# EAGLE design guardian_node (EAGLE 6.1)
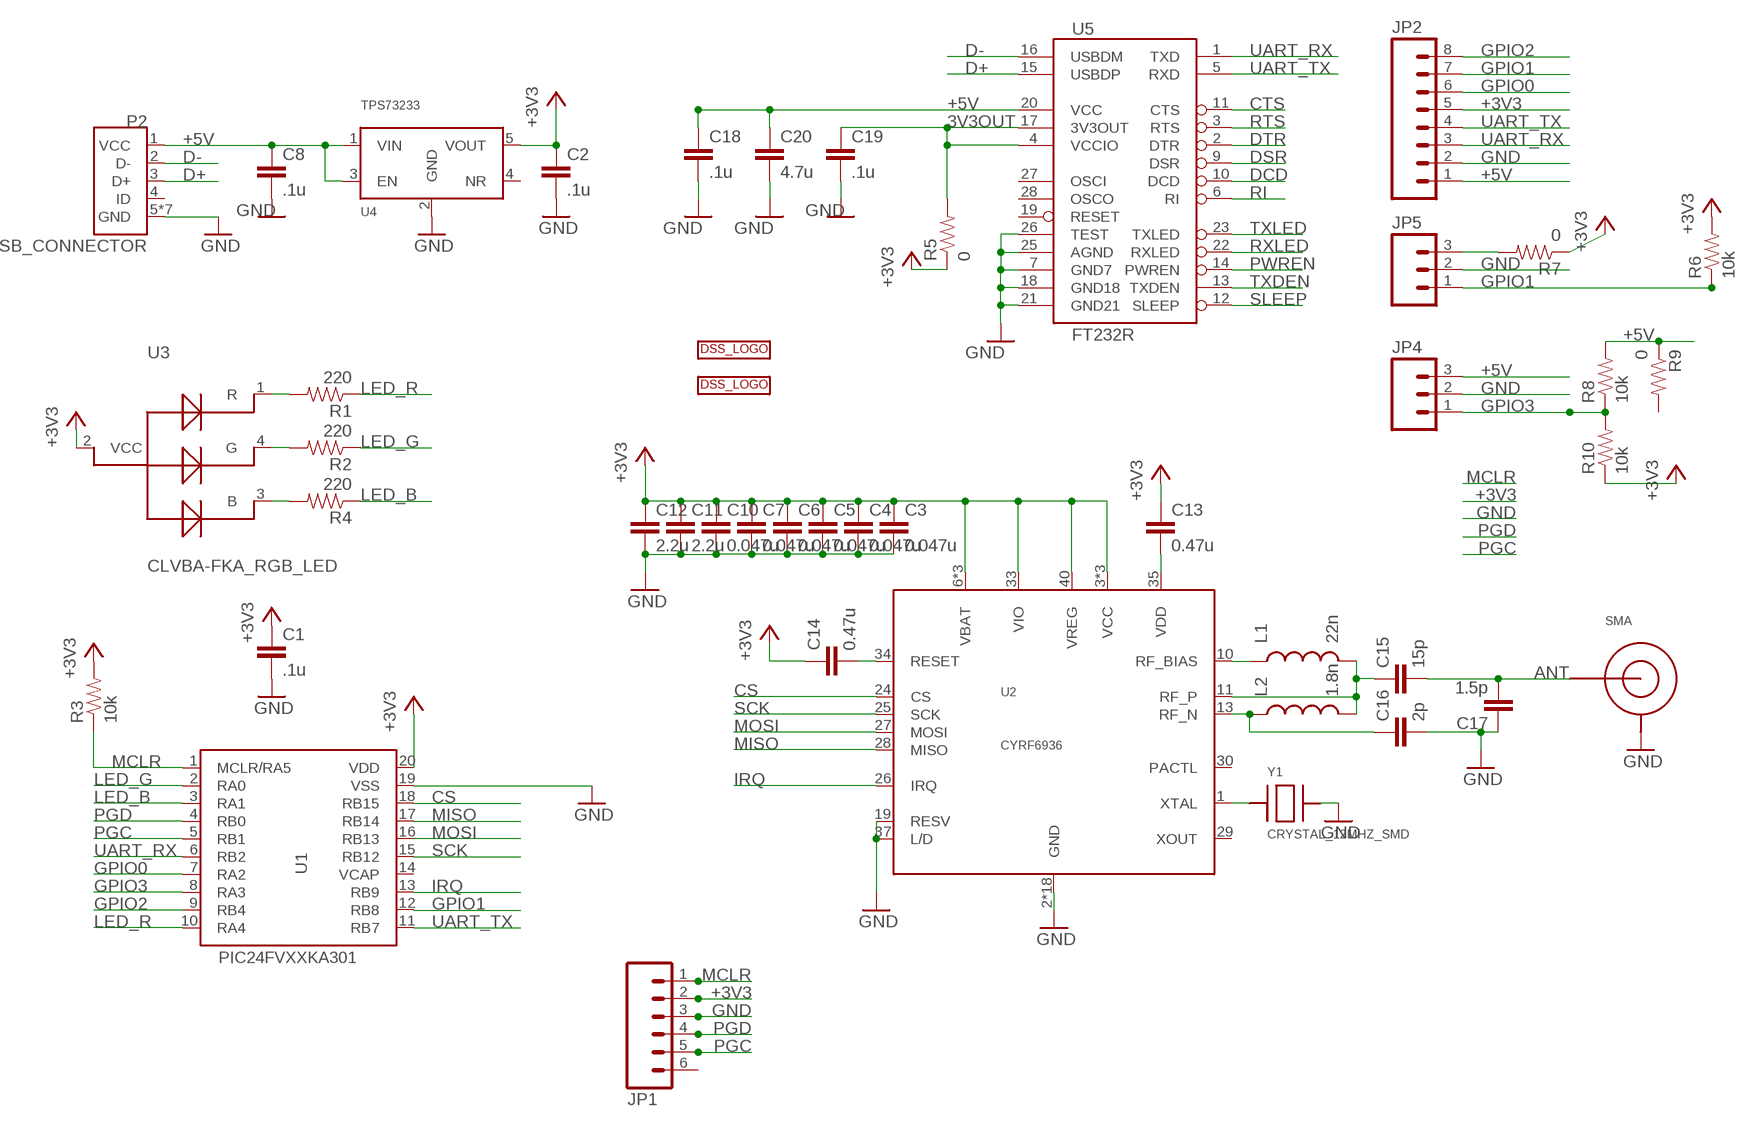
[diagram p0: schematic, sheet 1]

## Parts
C1  .1u  CAP0603-CAP  [0603-CAP]
C2  .1u  CAP0603-CAP  [0603-CAP]
C3  0.047u  CAP0402-CAP  [0402-CAP]
C4  0.047u  CAP0402-CAP  [0402-CAP]
C5  0.047u  CAP0402-CAP  [0402-CAP]
C6  0.047u  CAP0402-CAP  [0402-CAP]
C7  0.047u  CAP0402-CAP  [0402-CAP]
C8  .1u  CAP0603-CAP  [0603-CAP]
C10  0.047u  CAP0402-CAP  [0402-CAP]
C11  2.2u  CAP0402-CAP  [0402-CAP]
C12  2.2u  CAP0402-CAP  [0402-CAP]
C13  0.47u  CAP0402-CAP  [0402-CAP]
C14  0.47u  CAP0402-CAP  [0402-CAP]
C15  15p  CAP0402-CAP  [0402-CAP]
C16  2p  CAP0402-CAP  [0402-CAP]
C17  1.5p  CAP0402-CAP  [0402-CAP]
C18  .1u  CAP0603-CAP  [0603-CAP]
C19  .1u  CAP0603-CAP  [0603-CAP]
C20  4.7u  CAP0603-CAP  [0603-CAP]
JP1  M06SIP  [1X06]
JP2  M081X08  [1X08]
JP4  M03PTH  [1X03]
JP5  M03PTH  [1X03]
L1  22n  INDUCTOR0603  [0603]
L2  1.8n  INDUCTOR0402  [C0402]
P2  USB_CONNECTOR  [USB_MICRO]
R1  220  RESISTOR0402-RES  [0402-RES]
R2  220  RESISTOR0402-RES  [0402-RES]
R3  10k  RESISTOR0603-RES  [0603-RES]
R4  220  RESISTOR0402-RES  [0402-RES]
R5  0  RESISTOR0603-RES  [0603-RES]
R6  10k  RESISTOR0603-RES  [0603-RES]
R7  0  RESISTOR0603-RES  [0603-RES]
R8  10k  RESISTOR0603-RES  [0603-RES]
R9  0  RESISTOR0603-RES  [0603-RES]
R10  10k  RESISTOR0603-RES  [0603-RES]
SMA  SMA_PTH  [SMA_PTH]
U1  PIC24FVXXKA301  [SSOP20]
U2  CYRF6936  [QFN40-6X6]
U3  CLVBA-FKA_RGB_LED  [PLCC-4]
U4  TPS73233  [SOT23-5]
U5  FT232R  FT232RLSSOP  [SSOP28DB]
U$1  DSSBOTTOM  [DSS_BOT]
U$2  DSSTOP  [DSS]
Y1  CRYSTAL_12MHZ_SMD  [SMD-4_5X3.2MM]

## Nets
3V3OUT: C19.1 R5.2 U5.4(VCCIO) U5.17(3V3OUT)
+3V3: C1.1 C2.1 C3.1 C4.1 C5.1 C6.1 C7.1 C10.1 C11.1 C12.1 C13.1 C14.1 JP1.2 JP2.5 R3.2 R5.1 R6.2 R7.1 R10.1 U1.20(VDD) U2.3(VCC) U2.6(VBAT) U2.7(VCC) U2.8(VBAT) U2.16(VCC) U2.33(VIO) U2.38(VBAT) U2.40(VREG) U3.2(VCC) U4.5(VOUT)
+5V: C8.1 C18.1 C20.1 JP2.1 JP4.3 P2.1(VCC) R8.2 R9.1 U4.1(VIN) U4.3(EN) U5.20(VCC)
ANT: C15.2 C17.2 SMA.PIN(CENTER)
CS: U1.18(RB15) U2.24(CS)
CTS: U5.11(CTS)
D+: P2.3(D+) U5.15(USBDP)
D-: P2.2(D-) U5.16(USBDM)
DCD: U5.10(DCD)
DSR: U5.9(DSR)
DTR: U5.2(DTR)
GND: C1.2 C2.2 C3.2 C4.2 C5.2 C6.2 C7.2 C8.2 C10.2 C11.2 C12.2 C16.2 C17.1 C18.2 C19.2 C20.2 JP1.3 JP2.2 JP4.2 JP5.2 P2.5(GND) P2.GND1(GND) P2.GND2(GND) P2.GND3(GND) P2.GND4(GND) P2.GND5(GND) P2.GND6(GND) SMA.GND1(SHIELD) SMA.GND2(SHIELD) SMA.GND3(SHIELD) SMA.GND4(SHIELD) U1.19(VSS) U2.2(GND) U2.4(GND) U2.5(GND) U2.9(GND) U2.12(GND) U2.14(GND) U2.15(GND) U2.17(GND) U2.18(GND) U2.19(RESV) U2.20(GND) U2.21(GND) U2.22(GND) U2.23(GND) U2.31(GND) U2.32(GND) U2.36(GND) U2.37(L/D) U2.39(GND) U2.EXP(GND) U4.2(GND) U5.7(GND7) U5.18(GND18) U5.21(GND21) U5.25(AGND) U5.26(TEST) Y1.P$3
GPIO0: JP2.6 U1.7(RA2)
GPIO1: JP2.7 JP5.1 R6.1 U1.12(RB8)
GPIO2: JP2.8 U1.9(RB4)
GPIO3: JP4.1 R8.1 R10.2 U1.8(RA3)
IRQ: U1.13(RB9) U2.26(IRQ)
LED_B: R4.1 U1.3(RA1)
LED_G: R2.1 U1.2(RA0)
LED_R: R1.1 U1.10(RA4)
MCLR: JP1.1 R3.1 U1.1(MCLR/RA5)
MISO: U1.17(RB14) U2.28(MISO)
MOSI: U1.16(RB13) U2.27(MOSI)
N$1: R1.2 U3.1(R)
N$2: R2.2 U3.4(G)
N$3: R4.2 U3.3(B)
N$4: JP5.3 R7.2
N$5: L1.1 U2.10(RF_BIAS)
N$6: C15.1 L1.2 L2.2 U2.11(RF_P)
N$7: C13.2 U2.35(VDD)
N$8: C14.2 U2.34(RESET)
N$9: C16.1 L2.1 U2.13(RF_N)
N$10: U2.1(XTAL) Y1.P$1
PGC: JP1.5 U1.5(RB1)
PGD: JP1.4 U1.4(RB0)
PWREN: U5.14(PWREN)
RI: U5.6(RI)
RTS: U5.3(RTS)
RXLED: U5.22(RXLED)
SCK: U1.15(RB12) U2.25(SCK)
SLEEP: U5.12(SLEEP)
TXDEN: U5.13(TXDEN)
TXLED: U5.23(TXLED)
UART_RX: JP2.3 U1.6(RB2) U5.1(TXD)
UART_TX: JP2.4 U1.11(RB7) U5.5(RXD)
Unconnected: JP1.6 P2.4(ID) R9.2 U1.14(VCAP) U2.29(XOUT) U2.30(PACTL) U4.4(NR) U5.19(RESET) U5.27(OSCI) U5.28(OSCO)

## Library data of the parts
C1-C8 C10-C20 = SparkFun-Passives:CAP: Capacitor
JP1 = SparkFun-Connectors:M06: Header 6 Standard 6-pin 0.1" header. Use with straight break away headers (SKU : PRT-00116), right angle break away headers (PRT-00553), swiss pins (PRT-00743), machine pins (PRT-00117), and female headers (PRT-00115). Molex polarized connector foot print use with SKU : PRT-08094 with associated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
JP2 = SparkFun-Connectors:M08: Header 8 Standard 8-pin 0.1" header. Use with straight break away headers (SKU : PRT-00116), right angle break away headers (PRT-00553), swiss pins (PRT-00743), machine pins (PRT-00117), and female headers (PRT-00115).
JP4 JP5 = SparkFun-Connectors:M03: Header 3 Standard 3-pin 0.1" header. Use with straight break away headers (SKU : PRT-00116), right angle break away headers (PRT-00553), swiss pins (PRT-00743), machine pins (PRT-00117), and female headers (PRT-00115). Molex polarized connector foot print use with SKU : PRT-08232 with associated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
L1 L2 = SparkFun-Passives:INDUCTOR: Inductors
P2 = DSS:USB_CONNECTOR: USB Connector http://www.digikey.com/product-detail/en/10118192-0001LF/609-4613-1-ND/2785378
R1-R10 = SparkFun-Passives:RESISTOR: Resistor
SMA = DSS:SMA_PTH: SMA through-hole
U1 = DSS:PIC24FVXXKA301: PIC24FVXXKA301
U2 = DSS:CYRF6936: Cypress CYRF6936 2.4GHz DSSS radio. All N/C pins and the exposed pad are tied to ground.
U3 = DSS:CLVBA-FKA_RGB_LED
U4 = DSS:TPS73233: TI TPS73233 - fixed output http://www.ti.com/product/tps73233
U5 = SparkFun:FT232RL: USB UART FT232RL 4th Generation USB UART (USB <-> Serial) Controller. Spark Fun Electronics SKU : COM-00650
U$1 U$2 = DSS:DSS: DSS LOGO
Y1 = DSS:CRYSTAL_12MHZ_SMD: 12MHz crystal, SMD

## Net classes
2 VCC: width 0.406 mm, clearance 0.381 mm

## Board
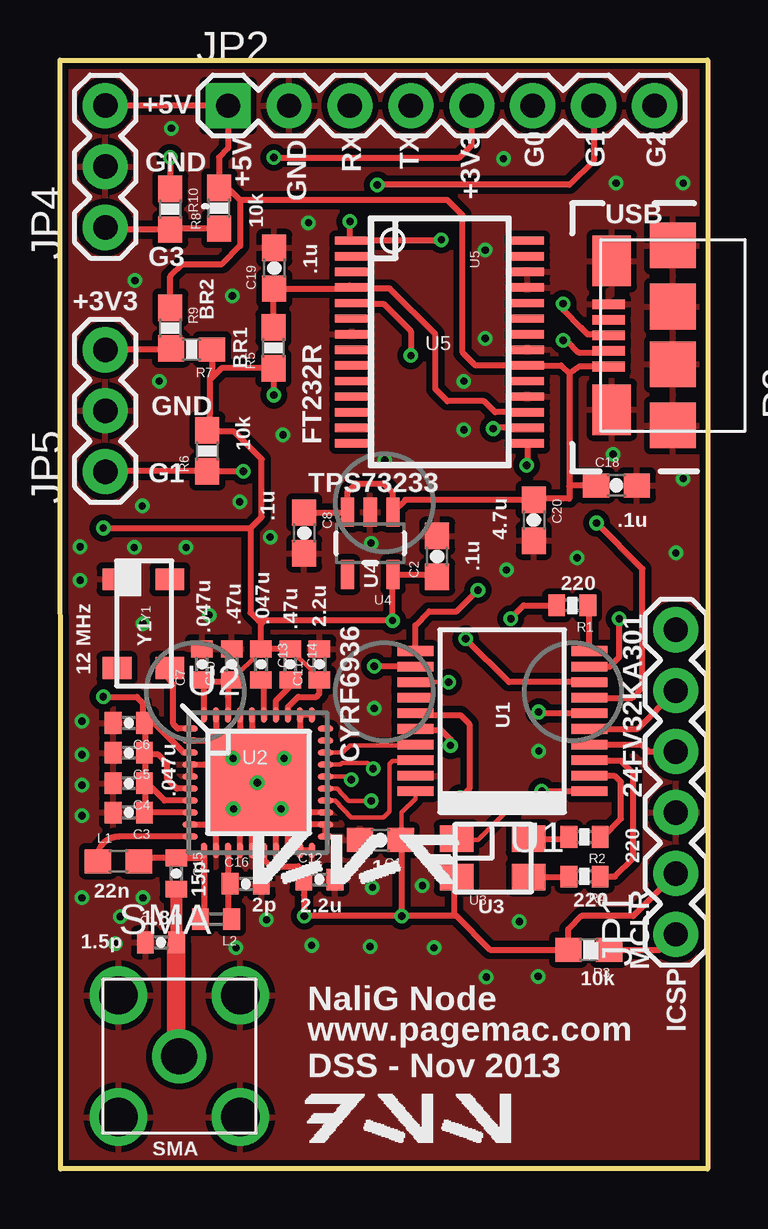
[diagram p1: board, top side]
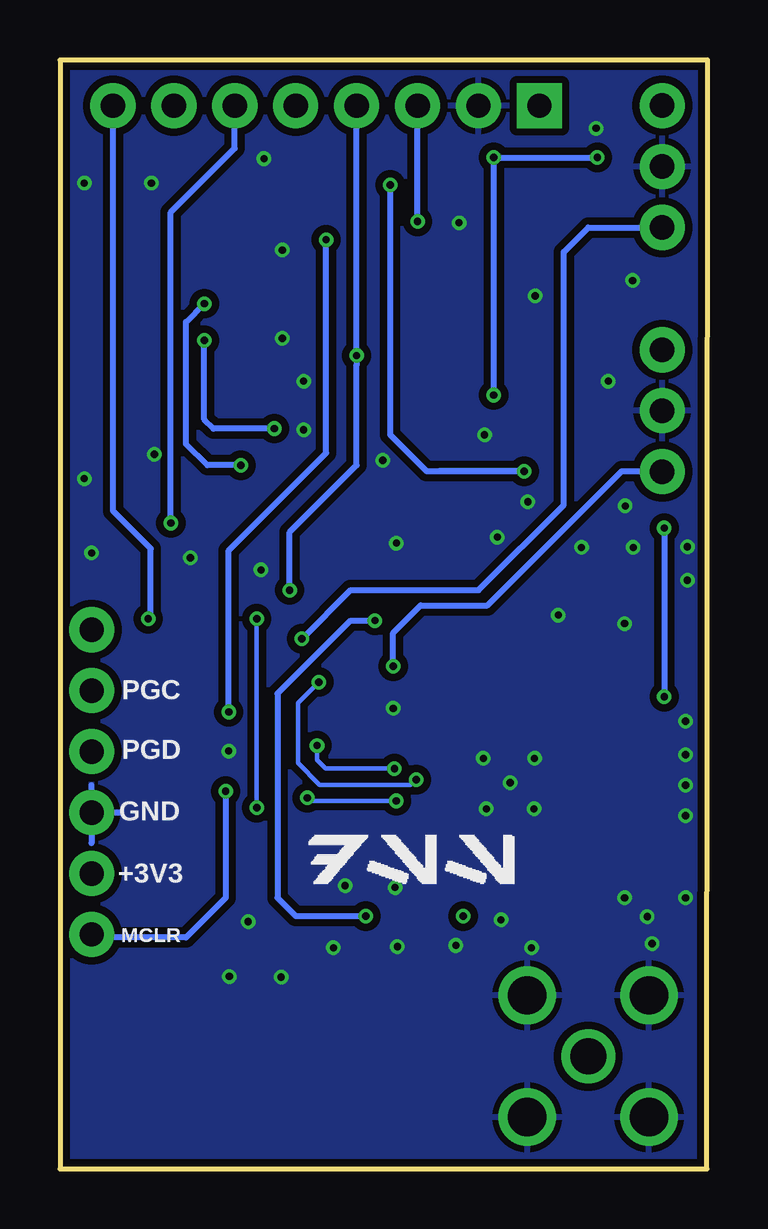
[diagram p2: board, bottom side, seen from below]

Size 27 x 46.23 mm. Coordinates in mm from the lower left corner, seen from the top.
Outline: 0,46.23 27,46.23 27,0 0.03,0 0,46.23
Copper layers (1*16): Top 0.035mm / dielectric 1.5mm / Bottom 0.035mm
Design rules: minimum track width 6mil, minimum drill 12mil, track to track 6mil, track to pad 6mil, pad to pad 6mil, via to via 6mil, smd to smd 0mil, copper to edge 10mil, drill to drill 10mil, minimum pad ring 10mil, minimum via ring 6mil, stop-mask expansion 2mil, vias tented up to drill 100mil, thermal gap 10mil
tRestrict: area 5.6,13.5 to 10.8,18.7; area 3.8,14.1 to 5.4,14.7; area 5.1,19.2 to 10.7,19.9

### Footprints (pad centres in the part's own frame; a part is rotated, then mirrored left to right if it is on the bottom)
0603-CAP = smd 1.1 x 1: 1 -0.85,0; 2 0.85,0
0402-CAP = smd 0.7 x 0.9: 1 -0.65,0; 2 0.65,0
1X06 = drill 1.016 pad 1.88: 1 0,0; 2 2.54,0; 3 5.08,0; 4 7.62,0; 5 10.16,0; 6 12.7,0
1X08 = drill 1.016 pad 1.88 square: 1 0,0 | drill 1.016 pad 1.88: 2 2.54,0; 3 5.08,0; 4 7.62,0; 5 10.16,0; 6 12.7,0; 7 15.24,0; 8 17.78,0
1X03 = drill 1.016 pad 1.88: 1 0,0; 2 2.54,0; 3 5.08,0
0603 = smd 1.1 x 1: 1 -0.85,0; 2 0.85,0
C0402 = smd 0.7 x 0.9: 1 -0.65,0; 2 0.65,0
USB_MICRO = smd 0.4 x 1.35: 1 -1.3,2.675; 2 -0.65,2.675; 3 0,2.675; 4 0.65,2.675; 5 1.3,2.675 | smd 1.9 x 1.9: GND1 -3.75,0; GND2 -1.2,0; GND3 1.2,0; GND4 3.75,0 | smd 2.1 x 1.6: GND5 -3.1,2.55; GND6 3.1,2.55
0402-RES = smd 0.7 x 0.9: 1 -0.65,0; 2 0.65,0
0603-RES = smd 1.1 x 1: 1 -0.85,0; 2 0.85,0
SMA_PTH = drill 1.6: GND1 2.54,2.54; GND2 -2.54,2.54; GND3 -2.54,-2.54; GND4 2.54,-2.54 | drill 1.5: PIN 0,0
SSOP20 = smd 0.4 x 1.5: 1 -2.925,-3.625; 2 -2.275,-3.625; 3 -1.625,-3.625; 4 -0.975,-3.625; 5 -0.325,-3.625; 6 0.325,-3.625; 7 0.975,-3.625; 8 1.625,-3.625; 9 2.275,-3.625; 10 2.925,-3.625; 11 2.925,3.625; 12 2.275,3.625; 13 1.625,3.625; 14 0.975,3.625; 15 0.325,3.625; 16 -0.325,3.625; 17 -0.975,3.625; 18 -1.625,3.625; 19 -2.275,3.625; 20 -2.925,3.625
QFN40-6X6 = smd 0.65 x 0.25: 1 -2.825,2.25; 2 -2.825,1.75; 3 -2.825,1.25; 4 -2.825,0.75; 5 -2.825,0.25; 6 -2.825,-0.25; 7 -2.825,-0.75; 8 -2.825,-1.25; 9 -2.825,-1.75; 10 -2.825,-2.25; 21 2.825,-2.25; 22 2.825,-1.75; 23 2.825,-1.25; 24 2.825,-0.75; 25 2.825,-0.25; 26 2.825,0.25; 27 2.825,0.75; 28 2.825,1.25; 29 2.825,1.75; 30 2.825,2.25 | smd 0.25 x 0.65: 11 -2.25,-2.825; 12 -1.75,-2.825; 13 -1.25,-2.825; 14 -0.75,-2.825; 15 -0.25,-2.825; 16 0.25,-2.825; 17 0.75,-2.825; 18 1.25,-2.825; 19 1.75,-2.825; 20 2.25,-2.825; 31 2.25,2.825; 32 1.75,2.825; 33 1.25,2.825; 34 0.75,2.825; 35 0.25,2.825; 36 -0.25,2.825; 37 -0.75,2.825; 38 -1.25,2.825; 39 -1.75,2.825; 40 -2.25,2.825 | smd 4.2 x 4.2: EXP 0,0
PLCC-4 = smd 1.4 x 1.1: 1 -1.524,0.812; 2 -1.524,-0.788; 3 1.476,-0.788; 4 1.476,0.812
SOT23-5 = smd 0.55 x 1.2: 1 -0.95,-1.3; 2 0,-1.3; 3 0.95,-1.3; 4 0.95,1.3; 5 -0.95,1.3
SSOP28DB = smd 0.348 x 1.397: 1 -4.225,-3.656; 2 -3.575,-3.656; 3 -2.925,-3.656; 4 -2.275,-3.656; 5 -1.625,-3.656; 6 -0.975,-3.656; 7 -0.325,-3.656; 8 0.325,-3.656; 9 0.975,-3.656; 10 1.625,-3.656; 11 2.275,-3.656; 12 2.925,-3.656; 13 3.575,-3.656; 14 4.225,-3.656; 15 4.225,3.656; 16 3.575,3.656; 17 2.925,3.656; 18 2.275,3.656; 19 1.625,3.656; 20 0.975,3.656; 21 0.325,3.656; 22 -0.325,3.656; 23 -0.975,3.656; 24 -1.625,3.656; 25 -2.275,3.656; 26 -2.925,3.656; 27 -3.575,3.656; 28 -4.225,3.656
SMD-4_5X3.2MM = smd 0.9 x 1.2: P$1 1.9,1.1; P$2 1.9,-1.1; P$3 -1.8,-1.1; P$4 -1.8,1.1

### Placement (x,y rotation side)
C1  13.36,13.72 180 top
C2  15.73,25.54 90 top
C3  2.87,14.86 180 top
C4  2.87,16.08 180 top
C5  2.87,17.35 180 top
C6  2.87,18.59 180 top
C7  5.92,21.03 90 top
C8  10.18,26.51 270 top
C10  7.16,21.03 90 top
C11  10.82,21.03 90 top
C12  10.82,12.06 0 top
C13  8.38,21.03 270 top
C14  9.6,21.03 270 top
C15  4.85,12.32 270 top
C16  7.75,11.89 0 top
C17  4.22,9.45 0 top
C18  23.2,28.49 0 top
C19  8.94,37.55 90 top
C20  19.76,27.04 270 top
JP1  25.68,9.78 90 top
JP2  7.01,44.32 0 top
JP4  1.89,39.25 90 top
JP5  1.89,29.07 90 top
L1  2.44,12.83 0 top
L2  6.5,10.41 180 top
P2  25.55,34.75 90 top
R1  21.36,23.49 180 top
R2  21.87,13.84 180 top
R3  22.05,9.14 180 top
R4  21.87,12.19 180 top
R5  8.9,34.23 90 top
R6  6.15,29.93 90 top
R7  5.49,34.16 180 top
R8  6.64,40.05 90 top
R9  4.6,35.05 270 top
R10  4.6,40 270 top
SMA  4.98,4.7 0 top
U1  18.44,18.67 90 top
U2  8.25,16.1 0 top
U3  18.06,12.95 0 top
U4  12.94,26.08 180 top
U5  15.83,34.47 270 top
U$1  7.9,11.68 0 top
U$2  10.06,0.89 0 top
Y1  3.48,22.78 270 top

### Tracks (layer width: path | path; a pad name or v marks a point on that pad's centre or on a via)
3V3OUT
  Top 0.254: U5.17 18.14,31.55 17.68,32 16.15,32 15.65,32.51 15.65,34.8 13.74,36.7 12.22,36.7 | 12.22,36.7 12.09,36.83 | R5.2 8.9,36.66 C19.1 12.12,36.7 U5.4 12.21,36.7 12.22,36.7
+3V3  (via drill 0.3)
  Top 0.178: U2.33 9.52,18.93 9.55,18.9 | 10.82,20.46 C14.1 | 8.38,21.6 C10.1 | U1.20 14.82,15.43 14.25,14.86 14.25,13.76 C1.1 | 10.19,12.32 C12.1
  Top 0.254: 3.58,14.86 U2.8 3.59,14.85 3.58,14.86 | U2.7 4.36,15.35 3.71,16 3.6,16 C4.1 3.57,16.13 3.58,16.13 | 3.45,17.41 C5.1 | U2.38 7.01,19.69 7.04,20.47 C10.1 7.1,20.32 5.99,20.32 6.01,20.31 U2.40 6.01,20.18 5.87,20.32 5.92,20.37 C7.1 | U2.16 8.51,12.91 8.79,12.62 9.93,12.62 10.19,12.32 | 10.82,20.46 C11.1 10.82,19.81 10.69,19.69 9.93,19.69 9.51,19.26 U2.33 | C14.1 C13.1 | C13.1 8.38,21.6 | v1.8,19.69 3.2,19.69 3.45,19.43 3.45,18.66 C6.1 3.57,18.54 3.58,18.54 | U2.6 4.87,15.85 4.47,16.26 4.47,16.89 4.09,17.27 3.45,17.27 3.45,17.29 C5.1 | U2.3 5.15,17.35 3.96,18.54 3.58,18.54 | 3.45,14.73 3.58,14.86 | C3.1 3.58,14.86 | 3.58,14.86 3.58,16.13 | 3.58,16.13 3.58,17.4 | 3.58,17.4 3.58,18.54 | C5.1 3.53,17.35 3.58,17.4 | 8.41,21.59 8.41,21.66 C13.1 | 16.51,12.19 U3.2 16.43,12.06 16.43,10.64 16.54,10.54 | 14.25,13.76 v14.25,10.54 | v14.25,10.54 v10.19,10.54 10.17,11.41 C12.1 | v1.8,26.72 7.95,26.72 | 6.25,32.89 6.25,33.02 6.34,33.11 R7.1 | 6.25,32.89 6.25,30.86 6.17,30.78 R6.2 6.2,30.78 6.25,30.73 7.26,30.73 8.41,29.59 8.41,27.18 7.95,26.72 | 6.25,32.89 6.73,33.38 R5.1 8.9,32.27 v8.92,32.26 | v8.92,42.16 16.66,42.16 17.17,42.67 JP2.5 | v4.6,42.16 R10.1 | C2.1 15.63,24.78 U4.5 13.87,24.76 v13.87,22.86 8.53,22.86 | 8.53,22.86 8.28,22.86 7.95,23.19 7.95,26.72 | C13.1 8.38,22.71 8.53,22.86 | 16.54,10.54 v14.25,10.54 | JP1.2 23.9,10.54 21.74,10.54 21.2,10 R3.2 17.93,9.14 16.54,10.54
  Bottom 0.254: v1.8,26.72 v1.8,19.69 | v8.92,32.26 v8.92,42.16 v4.6,42.16 | v14.25,10.54 17.17,10.54 17.93,11.3 17.93,19.81 14.88,22.86 v13.87,22.86
+5V
  Top 0.254: C8.1 11.97,27.36 U4.3 11.99,28.22 12.34,28.58 13.49,28.58 13.87,28.19 13.87,27.43 | 13.87,27.43 13.87,27.4 U4.1 14.4,27.89 C20.1 19.81,27.94 21.23,27.94 21.23,28.45 | P2.1 21.66,33.45 21.23,33.15 | 21.23,33.15 21.23,28.45 | 14,27.3 13.87,27.43 | 21.23,33.15 20.89,33.49 U5.20 17.33,33.49 16.79,34.04 16.79,39.75 16.15,40.39 7.52,40.39 | JP4.3 JP2.1 7.01,42.55 6.63,42.16 R8.2 7.01,40.89 7.52,40.39 | C18.1 21.28,28.49 21.23,28.45 | R9.1 4.6,37.21 5.11,37.72 6.76,37.72 7.52,38.48 7.52,40.39
ANT
  Top 0.254: 4.85,9.31 C17.2 | 4.85,4.83 arc90 SMA.PIN
  Top 0.508: C15.2 4.85,9.31
  Top 0.762: 4.85,9.31 4.85,4.83
CS
  Top 0.178: U2.24 11.47,15.35 12.14,14.66 13.49,14.66 13.74,14.91 13.74,16.89 13.87,17.02 14.79,17.02
  Top 0.254: 14.79,17.02 U1.18
D+  (via drill 0.3)
  Top 0.254: U5.15 19.48,29.36 v19.46,29.34 | v20.98,36.07 20.98,35.81 21.74,35.05 22,34.8 22.83,34.8 P2.3
  Bottom 0.254: v19.46,29.34 20.85,29.34 21.74,30.23 21.74,35.31 v20.98,36.07
D-  (via drill 0.3)
  Top 0.254: U5.16 18.09,30.9 v18.06,30.86 | v20.98,34.54 21.11,34.54 21.62,34.04 22.82,34.04 P2.2
  Bottom 0.254: v18.06,30.86 20.6,30.86 20.98,31.24 v20.98,34.54
GND  (via drill 0.3)
  Top 0.178: 6.51,14.28 6.86,14.63 v7.24,15.01 | v9.22,15.01 9.01,14.92 9.01,14.53 8.9,14.43 8.08,14.43 8.08,14.5 8.01,14.43 | 6.97,16.85 7.47,16.84 | 7.47,16.84 7.04,17.27 7.04,17.6 6.78,17.85 6.55,17.85 6.51,17.9 | 7.51,17.9 7.65,17.76 7.65,17.5 7.26,17.12 | 8.01,17.89 7.26,17.15 7.47,16.84 | 10.01,17.9 v9.35,17.12
  Top 0.254: U2.9 6.58,14.35 6.86,14.63 | U2.12 6.51,14.28 | U2.17 9.01,14.53 | U2.15 8.01,14.43 | U2.14 7.51,14.74 v7.24,15.01 | U2.2 6.55,17.85 | U2.39 6.51,17.9 | U2.37 7.51,17.9 | U2.36 8.01,17.89 | 7.26,17.15 6.97,16.85 U2.4 U2.5 | U2.31 U2.32 10.01,17.9 | U2.18 9.51,14.48 | 9.51,14.48 9.51,14.73 v9.22,15.01 9.37,14.86 9.93,14.86 | 9.72,14.27 10.01,13.98 U2.19 U2.20 | 9.72,14.27 9.51,14.48 | 9.72,14.27 9.81,14.35 U2.22 U2.21 | U2.23 9.94,14.85 9.93,14.86 | 9.8,14.99 9.93,14.86 | 7.47,16.84 7.49,16.84 v8.23,16.1 U2.EXP | 7.26,17.12 v9.35,17.12
  Bottom 0.254: JP1.3 24.46,14.86 | JP1.3 25.68,16 | JP1.3 25.68,13.59
  other vias: 7.49,27.81 10.49,9.32 6.22,23.09 15.6,9.22 0.91,18.67 7.34,9.22 2.31,9.4 0.91,11.3 2.51,10.52 25.68,25.68 0.91,17.27 0.91,16 0.91,14.73 3.45,11.3 17.78,8 19.15,10.31 0.84,25.93 3.45,22.73 21.56,25.48 12.93,9.27 3.1,25.91 19.94,8.03 3.43,27.64 4.14,32.84 12.97,26.09 9.3,30.61 8.76,26.34 18.62,24.97 16.84,30.81 23.19,41.1 13.54,29.54 25.98,41.1 25.98,28.78 19.96,17.42 13.03,11.73 17.73,38.3 3.12,37.03 7.19,36.4 4.65,43.38 23.06,29.79 18.49,42.11 10.36,39.45 16.84,32.84 17.73,34.62 13.11,19.2 15.11,11.81 5.26,25.91 0.84,24.54 7.21,17.12 8.61,10.39
  pour Top (isolate 0.254): -0.36,46.73 27.22,46.86 26.97,-0.03 0.03,-0.05
  pour Bottom (isolate 0.305): 0.03,-0.03 26.95,0.1 27.2,46.86 -0.33,46.68
GPIO0  (via drill 0.3)
  Top 0.254: U1.7 23.86,19.64 24.28,20.07 24.28,25.02 v22.38,26.92
  Bottom 0.254: v22.38,26.92 22.38,39.88 19.71,42.55 JP2.6
GPIO1  (via drill 0.3)
  Top 0.254: U1.12 13.12,20.94 v13.11,20.95 | JP5.1 1.91,29.08 R6.1 v7.65,29.08 | JP2.7 22.25,42.04 21.23,41.02 v13.23,41.02 | v7.65,29.08
  Bottom 0.254: v13.11,20.95 13.11,22.35 11.96,23.49 9.17,23.49 3.58,29.08 1.93,29.08 1.91,29.08 JP5.1 | v13.23,41.02 13.23,30.61 11.71,29.08 11.2,29.08 | 11.2,29.08 v7.65,29.08 11.2,29.08
GPIO2  (via drill 0.3)
  Top 0.254: U1.9 22.93,20.94 23.32,21.34 v23.32,22.94
  Bottom 0.254: v23.32,22.94 23.22,22.99 23.22,25.86 24.79,27.43 JP2.8
GPIO3  (via drill 0.3)
  Top 0.254: U1.8 18.72,20.29 v16.92,22.1 | R8.1 4.64,39.2 R10.2 2.02,39.16 1.93,39.24 JP4.1
  Bottom 0.254: v16.92,22.1 14.88,24.13 9.55,24.13 5.99,27.69 5.99,38.23 4.98,39.24 JP4.1
IRQ  (via drill 0.3)
  Top 0.178: U2.26 12.02,16.35 v12.14,16.23 | U1.13 v16.2,20.29 v16.21,20.3
  Bottom 0.178: v12.14,16.23 12.4,16 16.18,16 17.07,16.92 17.07,19.43 v16.21,20.3
LED_B
  Top 0.254: R4.1 23.14,12.19 23.9,12.95 23.9,16.51 23.39,17.02 22.09,17.02 U1.3
LED_G
  Top 0.254: R2.1 22.63,13.84 23.39,14.61 23.39,16.13 23.14,16.38 22.08,16.38 U1.2
LED_R
  Top 0.254: U1.10 22.07,23.44 R1.1
MCLR  (via drill 0.3)
  Top 0.254: U1.1 v20.1,15.74 v20.09,15.75 | R3.1 25.02,9.14 JP1.1
  Bottom 0.254: v20.09,15.75 20.09,11.3 21.74,9.65 25.55,9.65 JP1.1
MISO
  Top 0.178: U2.28 11.79,17.35 12.09,17.65 14.77,17.65
  Top 0.254: 14.77,17.65 U1.17
MOSI  (via drill 0.3)
  Top 0.178: U2.27 11.7,16.85 11.76,16.92 12.83,16.92 v13.06,16.69
  Top 0.254: U1.16 14.87,18.29 14.88,18.29 15.9,18.29 16.28,17.91 v16.28,17.65
  Bottom 0.178: v13.06,16.69 15.93,16.69 16.28,17.04 v16.28,17.65
N$1  (via drill 0.3)
  Top 0.178: v18.8,15.06 18.29,14.58 17.42,13.72 16.59,13.72 U3.1
  Top 0.254: R1.2 19.33,23.49 18.8,22.96 v18.8,22.94
  Bottom 0.178: v18.8,22.94 v18.8,15.06
N$2
  Top 0.254: U3.4 21.4,13.77 R2.2
N$3
  Top 0.254: U3.3 21.45,12.17 R4.2
N$4
  Top 0.254: R7.2 2.03,34.16 | 2.03,34.16 1.91,34.16 JP5.3 | 4.76,34.16 2.03,34.16
N$5
  Top 0.254: 1.42,12.7 1.42,12.74 L1.1 1.59,12.91 arc90 1.55,12.95 arc-90 2.45,13.85 U2.10
N$6
  Top 0.254: U2.11 6.01,12.06 | 6.01,12.06 6.01,10.55 5.87,10.41 L2.2 | 6.01,12.06 5.99,12.97 C15.1 3.18,12.97 L1.2
N$7
  Top 0.254: U2.35 8.51,20.26 C13.2
N$8
  Top 0.254: U2.34 9.01,19.52 9.55,20.07 9.55,20.33 C14.2
N$9
  Top 0.254: U2.13 7,11.5 C16.1 7.04,11.51 | L2.1 7.04,10.54 7.04,11.51 | 7.04,11.51 7.04,11.56
N$10
  Top 0.254: U2.1 4.91,18.35 4.72,18.54 4.72,20.19 4.34,20.7 4.6,20.83 4.58,20.94 Y1.P$1
PGC
  Top 0.254: U1.5 24.08,18.34 JP1.5
PGD
  Top 0.254: U1.4 24.24,17.69 24.54,17.4 JP1.4
SCK  (via drill 0.3)
  Top 0.178: U2.25 11.55,15.85 12.04,15.34 v12.98,15.34
  Top 0.254: U1.15 14.89,18.92 16.69,18.92 17.07,18.54 17.07,15.85 v16.69,15.47
  Bottom 0.178: v12.98,15.34 16.51,15.34 16.66,15.49 v16.69,15.47
UART_RX  (via drill 0.3)
  Top 0.254: U1.6 19.96,18.99 v19.96,19.05 | v15.9,38.73 15.61,38.7 U5.1 12.09,38.77 v12.09,39.5
  Bottom 0.254: v19.96,19.05 19.96,25.78 15.9,29.84 v15.9,38.73 | 12.09,44.45 JP2.3 v12.09,39.5
UART_TX  (via drill 0.3)
  Top 0.254: U1.11 14.82,22.66 15.39,23.24 16.54,23.24 v17.42,24.13 | U5.5 12.2,36.07 13.49,36.07 14.63,34.92 v14.63,33.91
  Bottom 0.254: v17.42,24.13 17.42,26.54 14.63,29.34 14.63,33.53 v14.63,33.91 JP2.4

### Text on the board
tDocu: B0 | B3 | B4 | B2 | B1
_tsilk: +5V | +5V | GND | RX | TX | +3V3 | G0 | G1 | G2 | GND | 10k | USB | G3 | .1u | +3V3 | BR2 | FT232R | U5 | BR1 | GND | 10k | G1 | TPS73233 | 4.7u | .1u | .1u | .1u | .047u | 220 | 12 MHz | .47u | U4 | Y1 | 2.2u | 24FV32KA301 | .047u | .47u | U1 | .047u | U2 | CYRF6936 | 220 | 15p | .1u | 220 | 22n | 1.8n | 2p | 2.2u | U3 | 1.5p | 10k | MCLR | NaliG Node | ICSP | www.pagemac.com | DSS - Nov 2013 | SMA
_bsilk: PGC | PGD | GND | +3V3 | MCLR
